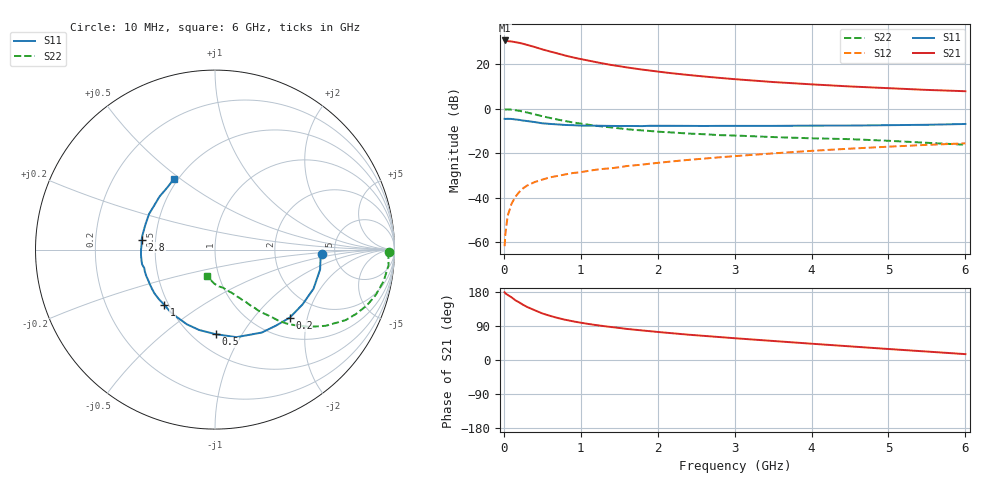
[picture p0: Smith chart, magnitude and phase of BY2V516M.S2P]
! SIEMENS Small Signal Semiconductors
! BFY420
! Si NPN RF SIEGET Grounded Emitter Transistor in MICRO-X
! VCE = 2.5 V  IC = 16 mA
! Common Emitter S-Parameters:  October  1996
# GHz  S  MA  R  50
!  f  S11  S21  S12  S22
! GHz  MAG  ANG  MAG  ANG  MAG  ANG  MAG  ANG
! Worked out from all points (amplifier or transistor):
!   36 points, 10 MHz to 6 GHz, reference 50 ohm
!   highest |S21| = 30.8 dB at 10 MHz (marker M1)
!   |S21| within 3 dB of that: start of sweep to 405.6 MHz
!   unconditionally stable (mu >= 1): 2.148 GHz to end of sweep
!   at 250 MHz: K = 0.26, MSG = 32.6 dB, |S12| = -35.9 dB
!   at 1.4 GHz: K = 0.87, MSG = 23.3 dB, |S12| = -26.8 dB
!   at 6 GHz: K = 1.08, MAG = 10.0 dB, |S12| = -15.6 dB
!   S11 on the Smith chart (normalised r, x): 10 MHz: 3.93, -0.29; 200 MHz: 1.41, -1.56; 500 MHz: 0.64, -0.78; 1 GHz: 0.47, -0.35; 2.8 GHz: 0.42, +0.06; 6 GHz: 0.48, +0.47
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0.01  0.5965 -2.3  34.75 178.8  0.0008 83.3  0.9696 -0.7
0.02  0.59 -4.6  34.37 176.0  0.0015 85.9  0.9663 -1.7
0.1  0.5906 -21.6  32.9 165.4  0.0072 81.1  0.9557 -10.6
0.15  0.5755 -32.1  31.82 157.6  0.0104 73.4  0.931 -15.7
0.2  0.5631 -42.4  30.68 152.0  0.0133 73.5  0.9017 -20.2
0.25  0.5428 -51.4  29.22 145.7  0.0161 68.8  0.8631 -24.6
0.3  0.5305 -60.6  27.73 140.2  0.0185 67.7  0.8276 -28.3
0.4  0.5024 -76.2  24.77 131.4  0.0223 62.9  0.7495 -34.5
0.5  0.4712 -89.6  21.88 122.9  0.0253 59.7  0.6807 -39.2
0.6  0.4565 -101.2  19.62 116.6  0.0285 58.2  0.6217 -42.9
0.7  0.4447 -110.7  17.67 110.9  0.0307 56.0  0.572 -46.0
0.8  0.4318 -119.3  15.87 106.1  0.0332 55.0  0.5286 -48.3
1  0.4181 -132.5  13.22 98.4  0.0373 54.5  0.4638 -51.5
1.1  0.4171 -138.7  12.22 95.1  0.0399 55.1  0.4379 -53.3
1.3  0.4134 -148.1  10.44 89.4  0.0443 55.1  0.3953 -55.6
1.6  0.4103 -159.2  8.561 82.0  0.0513 54.8  0.3473 -58.9
2.2  0.4136 -175.6  6.286 70.4  0.0655 53.9  0.2921 -64.4
2.8  0.4123 172.2  4.987 60.6  0.0805 51.3  0.2551 -69.3
3.5  0.4122 159.8  4.014 50.2  0.0989 47.5  0.2307 -74.8
4.5  0.4187 143.7  3.191 36.0  0.1263 40.1  0.2069 -83.6
5.5  0.4363 127.5  2.667 22.3  0.1538 31.3  0.1713 -97.7
6  0.4549 120.4  2.491 15.5  0.1666 26.6  0.1549 -107.5
